(* SV subscriber APDU *)
{attribute 'analysis' := '-33'}
{attribute 'no_assign'}
{attribute 'no_explicit_call' := 'Direct call not allowed for type FB_SVRXAPDU_IED_MUnn_LLN0_MSVCB01'}
FUNCTION_BLOCK FB_SVRXAPDU_IED_MUnn_LLN0_MSVCB01 EXTENDS FB_GseSvApduClass
VAR_OUTPUT
	RxData: ST_SVAPDU_IED_MUnn_LLN0_MSVCB01; (* Subscribed SV data in TwinCAT PLC host format (little endian) *)
END_VAR
VAR
	Asdu1: FB_SVRXASDU_IED_MUnn_LLN0_MSVCB01 := (index:=0, ipApdu:=THIS^.AddAsduToContainer(ipAsdu:=Asdu1)); (* Adds ASDU to APDU *)
END_VAR

{attribute 'analysis' := '-33'}
(* Converts received SV subscriber data from network (big-endian) to host (little-endian) byte order *)
METHOD FINAL OnSvSubscriberNetToHost
VAR_INPUT
	ipAdapter: I_GseAdapterClass; (* Network adapter interface pointer *)
	ipApdu: I_GseSvApduClass; (* APDU object interface pointer *)
END_VAR
VAR
END_VAR
RxData.Asdu1.nSmpCnt:= Asdu1.nSmpCnt; (* Get sample counter *)
RxData.Asdu1.eSmpSynch:= Asdu1.eSmpSynch; (* Get synchronization type: 0..2 *)
RxData.Asdu1.tRefrTm:= Asdu1.tRefrTm; (* Get refresh time stamp (optional) *)

(* Convert received SV data from network byte order to host byte order *)
NetToHostInt32(in:=Asdu1.Values.IED_MUnn_InnATCTR1_AmpSv_instMag_i, out:=RxData.Asdu1.IED_MUnn_InnATCTR1_AmpSv_instMag_i);
NetToHostQuality(in:=Asdu1.Values.IED_MUnn_InnATCTR1_AmpSv_q, out:=RxData.Asdu1.IED_MUnn_InnATCTR1_AmpSv_q);
NetToHostInt32(in:=Asdu1.Values.IED_MUnn_InnBTCTR2_AmpSv_instMag_i, out:=RxData.Asdu1.IED_MUnn_InnBTCTR2_AmpSv_instMag_i);
NetToHostQuality(in:=Asdu1.Values.IED_MUnn_InnBTCTR2_AmpSv_q, out:=RxData.Asdu1.IED_MUnn_InnBTCTR2_AmpSv_q);
NetToHostInt32(in:=Asdu1.Values.IED_MUnn_InnCTCTR3_AmpSv_instMag_i, out:=RxData.Asdu1.IED_MUnn_InnCTCTR3_AmpSv_instMag_i);
NetToHostQuality(in:=Asdu1.Values.IED_MUnn_InnCTCTR3_AmpSv_q, out:=RxData.Asdu1.IED_MUnn_InnCTCTR3_AmpSv_q);
NetToHostInt32(in:=Asdu1.Values.IED_MUnn_InnNTCTR4_AmpSv_instMag_i, out:=RxData.Asdu1.IED_MUnn_InnNTCTR4_AmpSv_instMag_i);
NetToHostQuality(in:=Asdu1.Values.IED_MUnn_InnNTCTR4_AmpSv_q, out:=RxData.Asdu1.IED_MUnn_InnNTCTR4_AmpSv_q);
NetToHostInt32(in:=Asdu1.Values.IED_MUnn_UnnATVTR1_VolSv_instMag_i, out:=RxData.Asdu1.IED_MUnn_UnnATVTR1_VolSv_instMag_i);
NetToHostQuality(in:=Asdu1.Values.IED_MUnn_UnnATVTR1_VolSv_q, out:=RxData.Asdu1.IED_MUnn_UnnATVTR1_VolSv_q);
NetToHostInt32(in:=Asdu1.Values.IED_MUnn_UnnBTVTR2_VolSv_instMag_i, out:=RxData.Asdu1.IED_MUnn_UnnBTVTR2_VolSv_instMag_i);
NetToHostQuality(in:=Asdu1.Values.IED_MUnn_UnnBTVTR2_VolSv_q, out:=RxData.Asdu1.IED_MUnn_UnnBTVTR2_VolSv_q);
NetToHostInt32(in:=Asdu1.Values.IED_MUnn_UnnCTVTR3_VolSv_instMag_i, out:=RxData.Asdu1.IED_MUnn_UnnCTVTR3_VolSv_instMag_i);
NetToHostQuality(in:=Asdu1.Values.IED_MUnn_UnnCTVTR3_VolSv_q, out:=RxData.Asdu1.IED_MUnn_UnnCTVTR3_VolSv_q);
NetToHostInt32(in:=Asdu1.Values.IED_MUnn_UnnNTVTR4_VolSv_instMag_i, out:=RxData.Asdu1.IED_MUnn_UnnNTVTR4_VolSv_instMag_i);
NetToHostQuality(in:=Asdu1.Values.IED_MUnn_UnnNTVTR4_VolSv_q, out:=RxData.Asdu1.IED_MUnn_UnnNTVTR4_VolSv_q);
END_METHOD

END_FUNCTION_BLOCK
